FUNCTION "ScambioSegnaliProfi" : VOID
TITLE =Scambio Segnali con Profibus
//Viene usata pe scambiare i seganli con il profibus
VERSION : 0.1

BEGIN
NETWORK
TITLE =Trasmissione Segnali
//Trasmette i seganli via profibus
// macchina in manuale
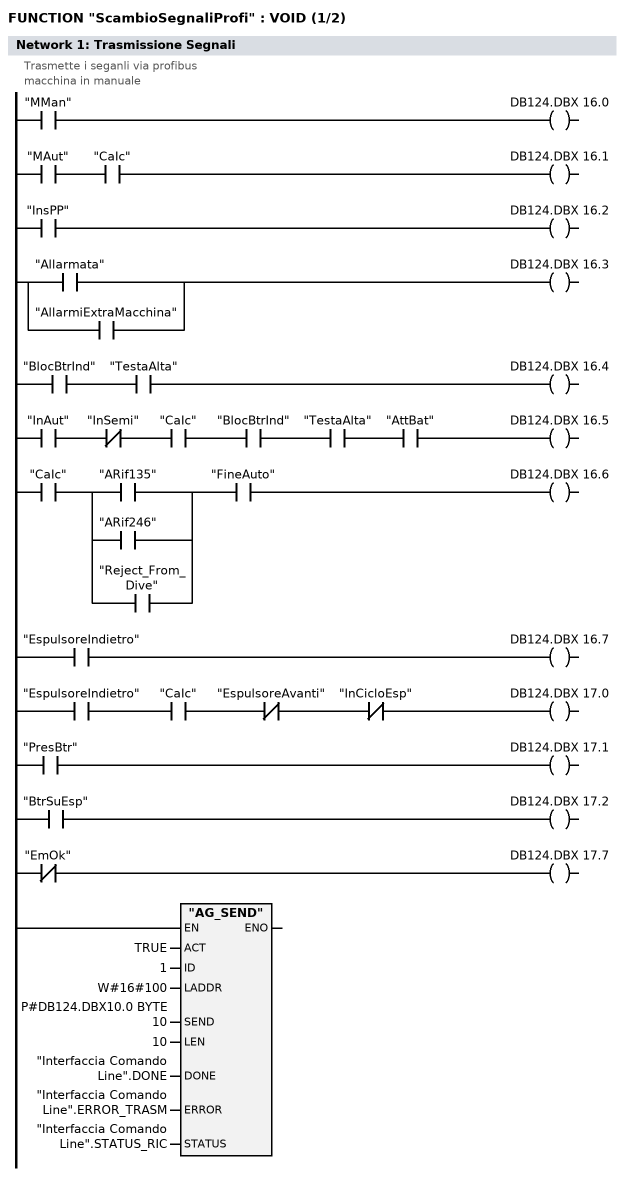
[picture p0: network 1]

      U     "MMan";
      =     DB124.DBX   16.0;

//------------------------------------

// macchina in automatico

      U     "MAut";
      U     "CaIc";
      =     DB124.DBX   16.1;

//-----------------------------------

// macchina inserita

      U     "InsPP";
      =     DB124.DBX   16.2;

//-----------------------------------

// macchina in avaria

      O     "Allarmata";
      O     "AllarmiExtraMacchina";
      =     DB124.DBX   16.3;

//----------------------------------

// macchina fuori ingombro

      U     "BlocBtrInd";
      U     "TestaAlta";
      =     DB124.DBX   16.4;

//----------------------------------

// Fine Ciclo
      U     "InAut";
      UN    "InSemi";
      U     "CaIc";
      U     "BlocBtrInd";
      U     "TestaAlta";
      U     "AttBat";
      =     DB124.DBX   16.5;

//----------------------------------

// Batteria da scartare

      U     "CaIc";
      U(    ;
      O     "ARif135";
      O     "ARif246";
      O     "Reject_From_Dive";
      )     ;
      U     "FineAuto";
      =     DB124.DBX   16.6;

//----------------------------------

// Espulsore indietro

      U     "EspulsoreIndietro";
      =     DB124.DBX   16.7;

//-----------------------------------

// Fine Ciclo espulsore

      U     "EspulsoreIndietro";
      U     "CaIc";
      UN    "EspulsoreAvanti";
      UN    "InCicloEsp";
      =     DB124.DBX   17.0;

//------------------------------------

// Presenza batteria sotto la macchina

      U     "PresBtr";
      =     DB124.DBX   17.1;


//------------------------------------
// Fotocellula espulsore 2

      U     "BtrSuEsp";
      =     DB124.DBX   17.2;

//------------------------------------
// Segnale emergenza in corso, attivo
// se sono in emergenza

      UN    "EmOk";
      =     DB124.DBX   17.7;



      CALL "AG_SEND" (
           ACT                      := TRUE,
           ID                       := 1,
           LADDR                    := W#16#100,
           SEND                     := P#DB124.DBX10.0 BYTE 10,
           LEN                      := 10,
           DONE                     := "Interfaccia Comando Line".DONE,
           ERROR                    := "Interfaccia Comando Line".ERROR_TRASM,
           STATUS                   := "Interfaccia Comando Line".STATUS_RIC);

NETWORK
TITLE =Ricezione Segnali
//Riceve i segnali via profibus
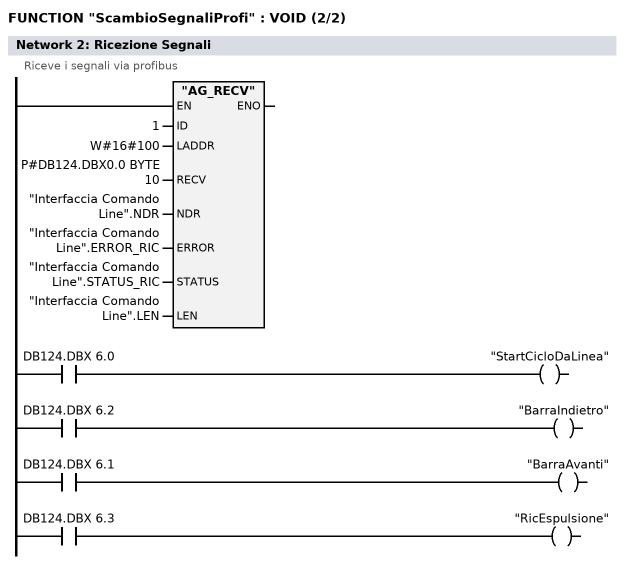
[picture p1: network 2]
      CALL "AG_RECV" (
           ID                       := 1,
           LADDR                    := W#16#100,
           RECV                     := P#DB124.DBX0.0 BYTE 10,
           NDR                      := "Interfaccia Comando Line".NDR,
           ERROR                    := "Interfaccia Comando Line".ERROR_RIC,
           STATUS                   := "Interfaccia Comando Line".STATUS_RIC,
           LEN                      := "Interfaccia Comando Line".LEN);


//----------------------------------------

// Ok start al ciclo

      U     DB124.DBX    6.0;
      =     "StartCicloDaLinea";

// Controllo barra indietro

      U     DB124.DBX    6.2;
      =     "BarraIndietro";

// Controllo che la barra sia avanti

      U     DB124.DBX    6.1;
      =     "BarraAvanti";

// Start ciclo espulsione

      U     DB124.DBX    6.3;
      =     "RicEspulsione";



END_FUNCTION

